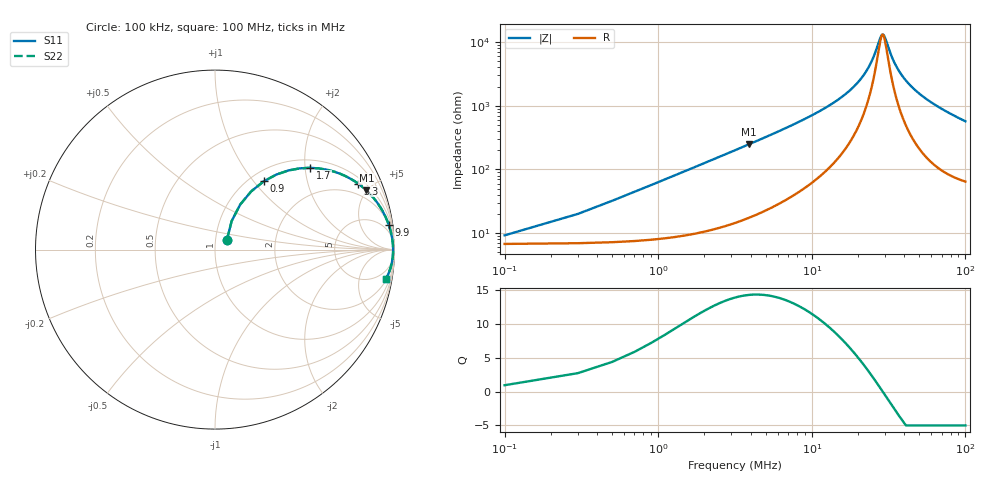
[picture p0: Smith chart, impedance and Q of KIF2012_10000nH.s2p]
!version-2
!date-12.2020
!Series
# MHz S RI R 50
!Freq ReS11 ImS11 ReS21 ImS21 ReS12 ImS12 ReS22 ImS22
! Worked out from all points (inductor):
!   501 points, 100 kHz to 100 MHz, reference 50 ohm
!   read as one part in series: L = 9.94 uH near 500 kHz
!   highest Q = 14.2 at 3.9 MHz (marker M1), where L = 10.1 uH
!   self-resonance near 28.9 MHz
!   S11 on the Smith chart (normalised r, x): 100 kHz: 1.14, +0.13; 900 kHz: 1.16, +1.13; 1.7 MHz: 1.19, +2.13; 3.3 MHz: 1.30, +4.17; 9.9 MHz: 2, +14; 100 MHz: 2, -11
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0.1  0.0665 0.0548  0.9335 -0.0548  0.9335 -0.0548  0.0665 0.0548
0.7  0.202 0.3248  0.798 -0.3248  0.798 -0.3248  0.202 0.3248
0.9  0.2712 0.3802  0.7288 -0.3802  0.7288 -0.3802  0.2712 0.3802
1.3  0.4101 0.4412  0.5899 -0.4412  0.5899 -0.4412  0.4101 0.4412
1.7  0.5304 0.4556  0.4696 -0.4556  0.4696 -0.4556  0.5304 0.4556
2.5  0.6988 0.4219  0.3012 -0.4219  0.3012 -0.4219  0.6988 0.4219
3.3  0.7969 0.3681  0.2031 -0.3681  0.2031 -0.3681  0.7969 0.3681
3.9  0.8434 0.33  0.1566 -0.33  0.1566 -0.33  0.8434 0.33
6.1  0.926 0.228  0.074 -0.228  0.074 -0.228  0.926 0.228
9.9  0.9684 0.1367  0.0316 -0.1367  0.0316 -0.1367  0.9684 0.1367
16.9  0.9873 0.0612  0.0127 -0.0612  0.0127 -0.0612  0.9873 0.0612
23.1  0.9915 0.0248  0.00851 -0.0248  0.00851 -0.0248  0.9915 0.0248
27.9  0.9924 0.00398  0.00758 -0.00398  0.00758 -0.00398  0.9924 0.00398
28.7  0.9925 0.000891  0.00754 -0.000891  0.00754 -0.000891  0.9925 0.000891
29.9  0.9925 -0.00358  0.00753 0.00358  0.00753 0.00358  0.9925 -0.00358
33.5  0.9922 -0.016  0.00777 0.016  0.00777 0.016  0.9922 -0.016
36.3  0.9918 -0.025  0.00822 0.025  0.00822 0.025  0.9918 -0.025
39.9  0.991 -0.0356  0.00904 0.0356  0.00904 0.0356  0.991 -0.0356
50.1  0.9874 -0.0626  0.0126 0.0626  0.0126 0.0626  0.9874 -0.0626
66.7  0.9785 -0.1001  0.0215 0.1001  0.0215 0.1001  0.9785 -0.1001
83.5  0.9667 -0.1335  0.0333 0.1335  0.0333 0.1335  0.9667 -0.1335
100  0.9526 -0.1629  0.0474 0.1629  0.0474 0.1629  0.9526 -0.1629
